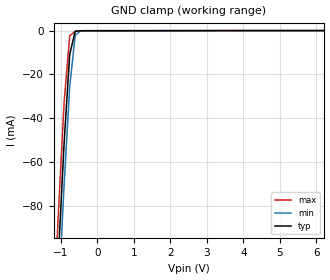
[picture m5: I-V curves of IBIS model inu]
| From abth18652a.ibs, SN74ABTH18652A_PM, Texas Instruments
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[Model]   inu
| input buffer with pullup resistor
| inu.abh (95186 ALEY)
| pad.abh (95272 ALEY)
Model_type   Input
Polarity   Non-Inverting
| Signals   OE#, TDI, TMS
Vinl = 0.8V
Vinh = 2.0V
| variable   typ   min   max
C_comp   5pF   NA   NA
| variable   typ   min   max
[Voltage range]   5.0V   4.5V   5.5V
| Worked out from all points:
|   GND clamp passes 1 mA (typ) near -0.62 V on its own axis
[gnd_clamp]
|   50C:5V:   100C:4.5V:weak   0C:5.5V:strong
|   Voltage   I(typ)   I(min)   I(max)
-5V       -1.557A    -1.574A    -1.54A
-1.212V   -153.4mA   -173.2mA   -133.8mA
-1.061V   -100.8mA   -120.6mA   -81.23mA
-909.1mV  -50.99mA   -70.2mA    -32.53mA
-757.6mV  -10.88mA   -25.7mA    -2.342mA
-606.1mV  -293.9uA   -2.13mA    -366.4uA
-454.5mV  -75.7uA    -77.64uA   -139.9uA
-303mV    -72.5uA    -44.19uA   -126.7uA
10V       3.501nA    3.715nA    3.45nA
